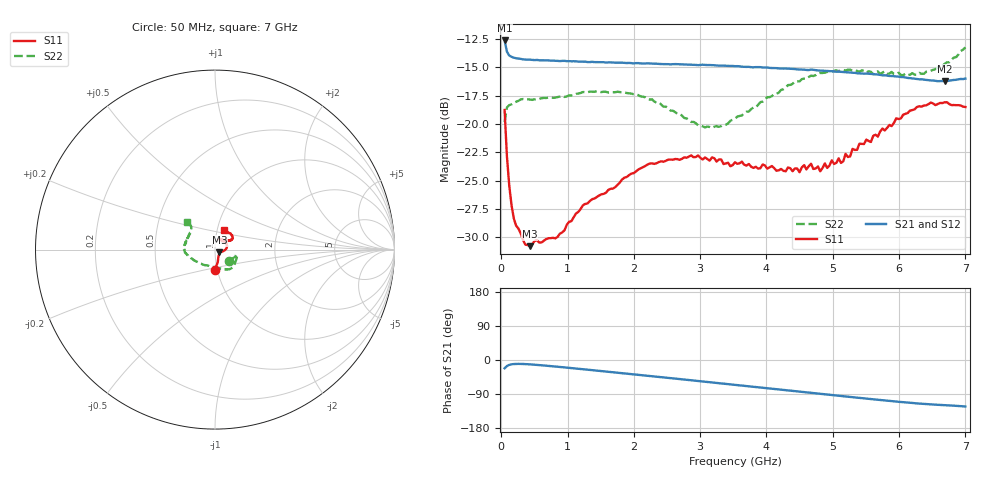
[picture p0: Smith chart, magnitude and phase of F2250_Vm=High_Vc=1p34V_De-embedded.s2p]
! Integrated Device Technology
! Corporate Headquarters
! 6024 Silver Creek Valley Road
! San Jose, CA 95138  USA
! Phone:  1-408-284-8200
! Toll Free:  1-800-223-1366
! Webpage:  http://www.idt.com/
! Timing and RF Division
! 515 Groton Road, Suite 102
! Westford, MA 01886-6024
! Device:  F2250
! Description: Voltage Variable RF Attenuator
! Frequency:  50.0 -  6000.00 MHz
! Package:  3x3 mm Thin QFN Plastic Package: 16 pin
! Ports:  2 RF, 3 DC
!  Pin  1  = GND
!  Pin  2  = NC
!  Pin  3  = RF1  = Port 1
!  Pin  4  = NC
!  Pin  5  = GND
!  Pin  6  = GND
!  Pin  7  = GND
!  Pin  8  = GND
!  Pin  9  = NC
!  Pin 10  = RF2  = Port 2
!  Pin 11  = NC
!  Pin 12  = GND
!  Pin 13  = GND
!  Pin 14  = VCNTRL
!  Pin 15  = VDD
!  Pin 16  = VMODE
! Vcntrl:  1.340 Volts
! Vmode:  +3.300 Volts
! Vdd:  +3.30  Volts
! Current:  1.333 mA
! Data:  The device was measured on a the F2250 evaluation board which has
!  individual transmission lines to the RF pins.  Data was collected
!  using a calibrated network analyzer.  The evaluation board was
!  de-embedded using a TRL calibration technique.
!  The reference plane is the edge of the package pin.
! Misc:  SN 10
!  Action Tracker AT0258
! Date Measured:  2014-11-26
! Date:  2015-10-15  MJV
! Note:
!  Integrated Device Technology supplies this data as a sample of measured
!  data at the package pin for this product.  Your particular data for this
!  product may vary.
!  Data was taken at 25 degrees C.
!  Integrated Device Technology reserves the right to change this data at anytime.
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# GHz S dB R 50
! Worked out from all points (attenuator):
!   201 points, 50 MHz to 7 GHz, reference 50 ohm
!   highest |S21| = -12.61 dB at 50 MHz (marker M1); lowest = -16.2 dB at 6.687 GHz (marker M2)
!   lowest |S11| = -30.8 dB at 432.2 MHz (marker M3), VSWR 1.06, Z = 52.5 - j1.56 ohm
!   |S11| at or under -10 dB: start of sweep to end of sweep
!   |S22| runs from -20.3 to -13.2 dB; largest |S21 - S12| = 0.00079
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0.05  -18.76 -91.1  -12.61 -21.9  -12.63 -21.9  -19.83 -38.0
0.08475  -22.84 -77.7  -13.60 -15.9  -13.60 -15.9  -18.53 -19.6
0.1195  -25.41 -70.9  -13.94 -13.0  -13.92 -12.9  -18.34 -14.6
0.189  -28.36 -56.8  -14.14 -10.7  -14.14 -10.7  -18.12 -12.9
0.36275  -30.66 -33.6  -14.30 -10.8  -14.30 -10.8  -17.84 -14.5
0.43225  -30.80 -31.0  -14.31 -11.5  -14.32 -11.5  -17.83 -15.7
0.84925  -29.98 -17.9  -14.42 -17.8  -14.44 -17.8  -17.62 -28.9
1.2315  -27.18 -13.8  -14.49 -24.3  -14.48 -24.3  -17.17 -38.6
1.857  -24.75 -0.7  -14.60 -35.3  -14.58 -35.3  -17.20 -51.0
2.37825  -23.36 12.5  -14.69 -44.6  -14.70 -44.6  -18.09 -62.7
3.07325  -22.95 34.2  -14.77 -57.3  -14.79 -57.3  -20.30 -96.0
3.525  -23.38 50.2  -14.89 -65.6  -14.89 -65.7  -19.53 -127.1
4.7065  -23.98 62.8  -15.21 -87.4  -15.23 -87.3  -15.76 -172.3
5.08875  -23.03 50.0  -15.37 -94.3  -15.35 -94.4  -15.32 179.3
5.1235  -23.44 50.2  -15.39 -95.0  -15.38 -95.0  -15.25 178.4
5.193  -22.64 45.4  -15.43 -96.2  -15.39 -96.3  -15.27 177.1
5.2625  -22.86 41.5  -15.45 -97.4  -15.43 -97.5  -15.20 176.2
5.29725  -22.20 41.1  -15.47 -98.0  -15.46 -98.1  -15.29 175.2
5.85325  -20.08 31.6  -15.75 -107.8  -15.74 -108.0  -15.54 160.6
6.27025  -18.49 33.3  -16.02 -114.5  -16.04 -114.5  -15.65 147.4
6.68725  -18.08 45.0  -16.23 -119.1  -16.24 -119.1  -14.68 135.8
7  -18.50 64.4  -15.98 -122.7  -16.01 -122.8  -13.22 135.6
